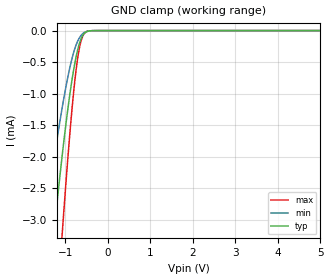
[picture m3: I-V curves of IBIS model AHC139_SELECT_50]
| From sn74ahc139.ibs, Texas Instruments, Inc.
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[Model]   AHC139_SELECT_50
Model_type  Input
Vinl=1.65
Vinh=3.85
| variable   typ   min   max
C_comp   0.74pF   0.55pF   0.88pF
[Temperature Range]   40   100   -40
| Ambient temperature   25   85   -40
[Voltage range]   5   4.5   5.5
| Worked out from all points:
|   GND clamp passes 1 mA (typ) near -0.89 V on its own axis
[GND Clamp]
| AHC139_SELECT_50
|   Voltage   I(typ)   I(min)   I(max)
-5.5V     -44.85mA   -29.94mA   -57.22mA
-1.52V    -5.007mA   -3.243mA   -7.831mA
-1.465V   -4.595mA   -2.969mA   -7.229mA
-1.265V   -3.18mA    -2.024mA   -5.105mA
-1.085V   -2.036mA   -1.259mA   -3.314mA
-1.06V    -1.889mA   -1.161mA   -3.077mA
-910mV    -1.081mA   -631.6uA   -1.752mA
-825mV    -697.7uA   -392.9uA   -1.103mA
-750mV    -420.6uA   -231.4uA   -630uA
-640mV    -145uA     -84.2uA    -184.3uA
-530mV    -29.43uA   -20.74uA   -28.38uA
5V        17.64nA    1.142nA    163.4nA
